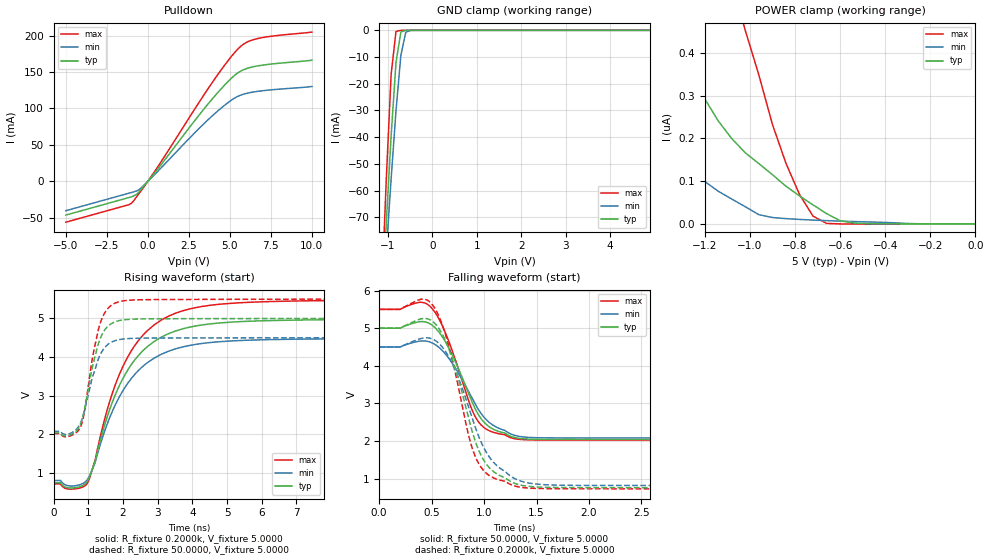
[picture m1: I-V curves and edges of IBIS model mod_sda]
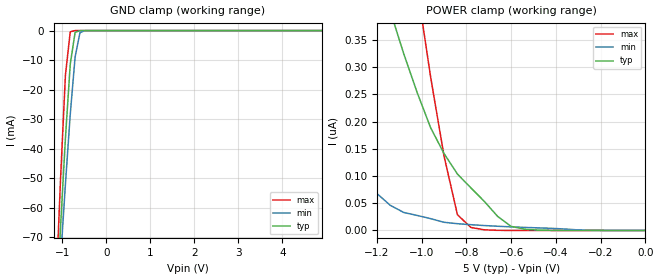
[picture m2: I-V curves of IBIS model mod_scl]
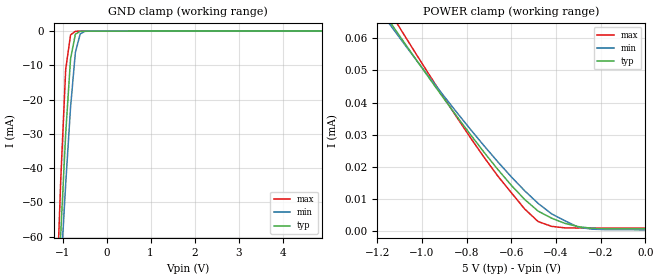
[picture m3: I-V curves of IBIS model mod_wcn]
| IBIS (I/O, Buffer, Information, Specification) Model, officially
| electronic behavioral standard for Buffer structures of digital pins.
[IBIS ver]  4.0
[File name] m24m04e_5d0_tssop8.ibs
[File Rev]  1.0
[Date]   13 Oct 2026
[Source]   CAD & Design Services (Catania) - STMicroelectronics
[Notes]
   (Note1)  This IBIS model includes the TSSOP8 package parasitic data
   (Note2)  This IBIS model has zero Notes and zero Warnings
[Disclaimer]
   Customers are solely responsible for all aspects of their
   own product designs or applications using this IBIS Model.
   STMicroelectronics assumes no liability for Custmer Designs
   and applications associated to this IBIS Model.
   In the use of this IBIS Model Customer shall not modify,
   disassemble, alter this Model in whole or in part.
   If Customers do not accept these terms, the IBIS Model
   may not be used. For any problems or modifications please
   contact STMicroelectronics (www.st.com).
[Copyright] (c) 2026 STMicroelectronics
|   Component M24M04E
[Component] M24M04E
[Manufacturer] STMicroelectronics
[Package]
| variable   typ   min   max
R_pkg   0.0   0.0   0.0
L_pkg   0.0H   0.0H   0.0H
C_pkg   0.0F   0.0F   0.0F
[Pin]  signal_name   model_name   R_pin   L_pin   C_pin
1   NC   NC   0.0   0.0   0.0
2   NC   NC   0.0   0.0   0.0
3   NC   NC   0.0   0.0   0.0
4   VSS   GND   0.0   0.0   0.0
5   SDA   mod_sda   0.0   0.0   0.0
6   SCL   mod_scl   0.0   0.0   0.0
7   WCN   mod_wcn   0.0   0.0   0.0
8   VCC   POWER   0.0   0.0   0.0
[Package Model]  182696_TSSOP8
[Define Package Model]  182696_TSSOP8
[Manufacturer]  STMicroelectronics
[OEM]  STMicroelectronics
[Description]  8 pin TSSOP package
[Number Of Pins]  8
[Pin Numbers]
|Pin Num   Terminal Name
1   | net1
2   | net2
3   | net3
4   | net4_GND
5   | net5
6   | net6
7   | net7
8   | net8_VDD
[Model Data]
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[End Model Data]
[End Package Model]
| Models and submodels in the file (3): mod_sda (I/O_open_drain), mod_scl (Input), mod_wcn (Input)
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|   Model mod_sda
[Model]   mod_sda
Model_type I/O_open_drain
Polarity   Inverting
Enable   Active-High
Vinl   =   1.500V
Vinh   =   3.500V
Vmeas  =   2.500V
Cref   =   30pF
Rref   =   500
Vref   =   5.000V
C_comp   4.636pF   4.427pF   4.856pF
[Temperature Range]  25.0000   85.0000   -40.0000
[Voltage Range]   5.0000V   4.5000V   5.5000V
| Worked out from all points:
|   slope of the pulldown table from 0 to 0.75 V, typ, clamps not added: 35.3 ohm
|   GND clamp passes 1 mA (typ) near -0.71 V on its own axis
|   rising waveform, R_fixture 0.2000k, V_fixture 5.0000: 20-80 % time 1.26ns typ, 1.27ns min, 1.26ns max; typ from 0.75 V to 4.97 V
|   rising waveform, R_fixture 50.0000, V_fixture 5.0000: 20-80 % time 426ps typ, 446ps min, 404ps max; typ from 2.04 V to 5 V
|   falling waveform, R_fixture 50.0000, V_fixture 5.0000: 20-80 % time 286ps typ, 313ps min, 261ps max; typ from 5 V to 2.04 V
|   falling waveform, R_fixture 0.2000k, V_fixture 5.0000: 20-80 % time 273ps typ, 314ps min, 242ps max; typ from 5 V to 0.752 V
[Pulldown]
|Voltage   I(typ)   I(min)   I(max)
-5V       -46.32mA   -40.32mA   -56.11mA
-1V       -21.32mA   -15.32mA   -30.1mA
-680mV    -17.9mA    -13.22mA   -21.04mA
-520mV    -13.92mA   -11.3mA    -16.25mA
760mV     21.55mA    17.37mA    25.35mA
2.84V     82.84mA    66.22mA    98.7mA
4.12V     118.2mA    93.82mA    142mA
5.08V     141.3mA    111.3mA    171.1mA
5.72V     152.1mA    118.8mA    186.5mA
6.2V      156.1mA    121.7mA    192.7mA
6.84V     159mA      124mA      196.7mA
10V       166.3mA    130.2mA    204.9mA
[GND_clamp]
|Voltage   I(typ)   I(min)   I(max)
-5V       -1.422A    -1.176A    -1.866A
-1.15V    -107.2mA   -111.7mA   -101.9mA
-1.04V    -72.5mA    -83.27mA   -56.29mA
-930mV    -39.66mA   -55.77mA   -16.56mA
-820mV    -12.07mA   -30.13mA   -402.8uA
-710mV    -609.6uA   -9.335mA   -4.14uA
-600mV    -10.22uA   -717.4uA   -32.48nA
-490mV    -151.4nA   -22.68uA   -140.4pA
4.9V      24.41pA    1.481nA    23.56pA
[POWER_clamp]
|Voltage   I(typ)   I(min)   I(max)
-4.98V    22.67uA    13.45uA    39.59uA
-1.8V     927nA      454.3nA    3.005uA
-1.62V    682nA      304.3nA    2.197uA
-1.38V    447.3nA    168.6nA    1.383uA
-1.14V    240.9nA    76.49nA    697.7nA
-1.02V    166.3nA    40.21nA    452.1nA
-900mV    115.3nA    15.06nA    232.9nA
-840mV    88.27nA    12.47nA    142nA
-780mV    65.71nA    10.63nA    69.1nA
-720mV    44.6nA     9.087nA    18.24nA
-540mV    2.332nA    5.661nA    40.22pA
0V        24.99pA    35.71pA    26.88pA
[Ramp]
| variable   typ   min   max
dV/dt_r   1.7772/0.4957n   1.4534/0.5134n   2.0879/0.4753n
dV/dt_f   1.7776/0.3030n   1.4537/0.3605n   2.0883/0.2757n
R_load = 50.0000
[Rising Waveform]
R_fixture= 0.2000k
V_fixture= 5.0000
V_fixture_min= 4.5000
V_fixture_max= 5.5000
|time   V(typ)   V(min)   V(max)
0s        749.7mV    806.9mV    717.9mV
530ps     612.3mV    663.3mV    582.8mV
970ps     776.1mV    823.2mV    729.1mV
1.2ns     1.308V     1.273V     1.336V
1.61ns    2.622V     2.413V     2.826V
2.02ns    3.478V     3.159V     3.794V
2.59ns    4.174V     3.77V      4.576V
3.3ns     4.597V     4.144V     5.049V
5.1ns     4.9V       4.413V     5.386V
10ns      4.975V     4.478V     5.473V
[Rising Waveform]
R_fixture= 50.0000
V_fixture= 5.0000
V_fixture_min= 4.5000
V_fixture_max= 5.5000
|time   V(typ)   V(min)   V(max)
0s        2.037V     2.077V     2.019V
430ps     1.97V      2.008V     1.946V
770ps     2.242V     2.278V     2.176V
880ps     2.586V     2.574V     2.527V
1.12ns    3.74V      3.466V     3.966V
1.32ns    4.414V     4.009V     4.799V
1.52ns    4.749V     4.288V     5.202V
1.81ns    4.92V      4.432V     5.405V
2.7ns     4.986V     4.489V     5.482V
10ns      4.997V     4.497V     5.497V
[Falling Waveform]
R_fixture= 50.0000
V_fixture= 5.0000
V_fixture_min= 4.5000
V_fixture_max= 5.5000
|time   V(typ)   V(min)   V(max)
0s        5V         4.5V       5.5V
390ps     5.173V     4.657V     5.688V
490ps     5.108V     4.626V     5.568V
570ps     4.896V     4.49V      5.248V
660ps     4.496V     4.216V     4.68V
870ps     3.144V     3.221V     2.938V
940ps     2.729V     2.866V     2.537V
1.08ns    2.326V     2.431V     2.24V
1.32ns    2.077V     2.132V     2.05V
10ns      2.038V     2.078V     2.02V
[Falling Waveform]
R_fixture= 0.2000k
V_fixture= 5.0000
V_fixture_min= 4.5000
V_fixture_max= 5.5000
|time   V(typ)   V(min)   V(max)
0s        5V         4.5V       5.5V
410ps     5.254V     4.733V     5.773V
510ps     5.18V      4.71V      5.615V
590ps     4.9V       4.537V     5.179V
680ps     4.327V     4.154V     4.354V
850ps     2.638V     2.928V     2.181V
930ps     1.888V     2.26V      1.503V
1.08ns    1.21V      1.467V     1.032V
1.34ns    833.5mV    944.4mV    775.1mV
10ns      752.1mV    809.5mV    720mV
|   Model mod_scl
[Model]   mod_scl
Model_type Input
Vinl   =   1.500V
Vinh   =   3.500V
C_comp   3.062pF   2.954pF   3.207pF
[Temperature Range]  25.0000   85.0000   -40.0000
[Voltage Range]   5.0000V   4.5000V   5.5000V
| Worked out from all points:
|   GND clamp passes 1 mA (typ) near -0.71 V on its own axis
[GND_clamp]
|Voltage   I(typ)   I(min)   I(max)
-5V       -1.288A    -1.088A    -1.629A
-1.15V    -97.84mA   -103.9mA   -89.96mA
-1.04V    -66.36mA   -77.58mA   -50.08mA
-930mV    -36.57mA   -52.12mA   -15.17mA
-820mV    -11.39mA   -28.35mA   -400.5uA
-710mV    -605.6uA   -8.962mA   -4.139uA
-600mV    -10.22uA   -713uA     -32.48nA
-490mV    -151.4nA   -22.67uA   -140.4pA
4.9V      24.41pA    781pA      23.56pA
[POWER_clamp]
|Voltage   I(typ)   I(min)   I(max)
-4.98V    22.67uA    13.45uA    39.59uA
-1.86V    1.263uA    382.3nA    3.336uA
-1.56V    907nA      199.3nA    1.965uA
-1.14V    402.8nA    46.2nA     727.7nA
-1.08V    324.5nA    33.1nA     580.5nA
-1.02V    253.3nA    27.61nA    447.1nA
-960mV    188.8nA    21.75nA    282.3nA
-900mV    141.3nA    15.06nA    136.9nA
-840mV    103.6nA    12.47nA    28.93nA
-780mV    78.3nA     10.63nA    5.549nA
-600mV    7.55nA     6.641nA    82.93pA
0V        24.99pA    35.71pA    26.88pA
|   Model mod_wcn
[Model]   mod_wcn
Model_type Input
Vinl   =   1.500V
Vinh   =   3.500V
C_comp   3.062pF   2.954pF   3.207pF
[Temperature Range]  25.0000   85.0000   -40.0000
[Voltage Range]   5.0000V   4.5000V   5.5000V
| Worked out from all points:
|   GND clamp passes 1 mA (typ) near -0.71 V on its own axis
[GND_clamp]
|Voltage   I(typ)   I(min)   I(max)
-5V       -1.278A    -1.078A    -1.619A
-1.15V    -89.34mA   -95.35mA   -81.49mA
-1.04V    -58.44mA   -69.42mA   -42.62mA
-930mV    -29.87mA   -44.63mA   -11.17mA
-820mV    -8.118mA   -22.27mA   -1.101mA
-710mV    -875.5uA   -6.209mA   -37.4uA
-600mV    -38.55uA   -792.1uA   -12.65uA
-490mV    -9.651uA   -47.19uA   -9.595uA
4.9V      13.25uA    4.492uA    21.54uA
[POWER_clamp]   |  NEWWWWW
|Voltage   I(typ)   I(min)   I(max)
-4.98V    513.1uA    484.3uA    552.1uA
-1.14V    64.79uA    63.99uA    67.87uA
-1.08V    58.76uA    58.34uA    61.13uA
-900mV    41.07uA    41.88uA    41.36uA
-720mV    24.35uA    26.38uA    22.77uA
-600mV    14.24uA    16.86uA    11.94uA
-540mV    9.809uA    12.51uA    6.844uA
-480mV    6.196uA    8.597uA    2.949uA
-420mV    4.002uA    5.356uA    1.454uA
-300mV    1.36uA     1.18uA     935.5nA
-240mV    851.3nA    577.4nA    935.4nA
0V        750.3nA    340nA      935.3nA
